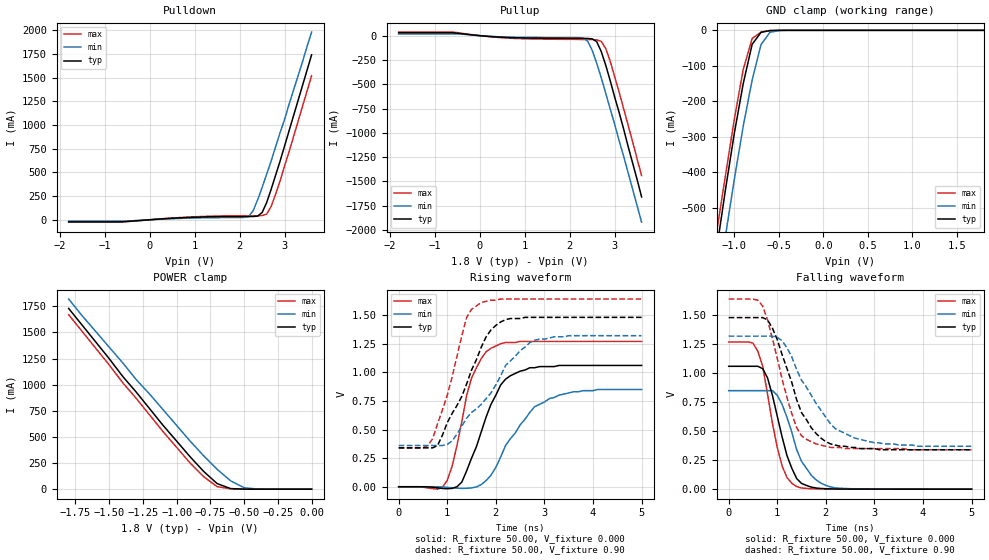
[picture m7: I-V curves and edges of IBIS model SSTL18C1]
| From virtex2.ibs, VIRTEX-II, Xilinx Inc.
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|   Model SSTL18C1
[Model]   SSTL18C1
Model_type   I/O
Polarity   Non-Inverting
Enable   Active-Low
Vinh = 1.025v
Vinl = 0.775v
Vmeas =   0.90V
Cref =  30.00pF
Rref =  50.00
Vref =   0.90V
C_comp   7.00pF   6.00pF   8.00pF
[Temperature Range]   25.00   100.00   0.000
[Voltage Range]   1.80V   1.70V   1.90V
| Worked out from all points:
|   slope of the pulldown table from 0 to 0.27 V, typ, clamps not added: 29.1 ohm
|   slope of the pullup table from 0 to 0.27 V, typ, clamps not added: 26.6 ohm
|   GND clamp passes 1 mA (typ) near -0.61 V on its own axis
|   POWER clamp passes 1 mA (typ) near -0.51 V on its own axis
|   rising waveform, R_fixture 50.00, V_fixture 0.000: 20-80 % time 588ps typ, 760ps min, 432ps max; typ from 0 V to 1.06 V
|   rising waveform, R_fixture 50.00, V_fixture 0.90: 20-80 % time 726ps typ, 1.04ns min, 496ps max; typ from 0.34 V to 1.48 V
|   falling waveform, R_fixture 50.00, V_fixture 0.000: 20-80 % time 396ps typ, 471ps min, 348ps max; typ from 1.06 V to 0 V
|   falling waveform, R_fixture 50.00, V_fixture 0.90: 20-80 % time 616ps typ, 791ps min, 492ps max; typ from 1.48 V to 0.34 V
[Pulldown]
| voltage   I(typ)   I(min)   I(max)
-1.8V     -22.43mA   -14.43mA   -25.5mA
-700mV    -22.43mA   -14.43mA   -25.5mA
900mV     24.93mA    17.53mA    29.31mA
2.2V      34.25mA    34.8mA     41.86mA
2.3V      34.66mA    95.09mA    41.97mA
2.4V      38.31mA    210mA      42.34mA
2.5V      76.54mA    340mA      44.73mA
2.6V      180mA      480mA      59.03mA
2.7V      320mA      620mA      140mA
2.9V      620mA      920mA      410mA
3V        780mA      1.06A      570mA
3.6V      1.74A      1.98A      1.52A
[Pullup]
| voltage   I(typ)   I(min)   I(max)
-1.8V     29.35mA    17.06mA    36.57mA
-600mV    29.35mA    17.06mA    36.57mA
600mV     -18.84mA   -14.55mA   -24.59mA
2.2V      -28.12mA   -21.34mA   -38.85mA
2.4V      -29.08mA   -55.84mA   -39.41mA
2.5V      -33.23mA   -150mA     -40.04mA
2.6V      -60.46mA   -280mA     -43.55mA
2.7V      -160mA     -430mA     -57.58mA
2.8V      -300mA     -590mA     -130mA
2.9V      -460mA     -750mA     -260mA
3.1V      -790mA     -1.08A     -580mA
3.6V      -1.66A     -1.92A     -1.44A
[GND_clamp]
| voltage   I(typ)   I(min)   I(max)
-1.8V     -1.65A     -1.74A     -1.6A
-1.2V     -620mA     -740mA     -570mA
-1.1V     -450mA     -580mA     -410mA
-1V       -290mA     -420mA     -250mA
-900mV    -150mA     -270mA     -110mA
-800mV    -39.2mA    -140mA     -23mA
-700mV    -5.61mA    -40.17mA   -4.8mA
-600mV    -750uA     -5.57mA    -620uA
-500mV    -57.3uA    -660uA     -36.33uA
1.8V      30.92pA    98.88nA    20.22pA
[POWER_clamp]
| voltage   I(typ)   I(min)   I(max)
-1.8V     1.73A      1.82A      1.67A
-1.7V     1.57A      1.66A      1.51A
-1.4V     1.08A      1.21A      1.02A
-1.3V     930mA      1.05A      870mA
-1.1V     610mA      760mA      550mA
-900mV    310mA      460mA      250mA
-800mV    170mA      320mA      120mA
-700mV    53.56mA    190mA      24.17mA
-600mV    5.5mA      79.88mA    3.5mA
-500mV    490uA      13.45mA    470uA
-400mV    34.21uA    820uA      28.36uA
0V        30.92pA    1.07nA     28.99pA
[Ramp]
| variable   typ   min   max
dV/dt_r   0.64/0.57n   0.51/0.80n   0.76/0.43n
dV/dt_f   0.64/0.76n   0.50/1.09n   0.72/0.59n
R_load = 50.00
[Rising Waveform]
R_fixture = 50.00
V_fixture = 0.000
| time   V(typ)   V(min)   V(max)
0s        0V         0V         0V
800ps     -9.52mV    -300uV     -21.25mV
1ns       -17.24mV   -5.02mV    56.09mV
1.3ns     40.76mV    -14.5mV    570mV
1.5ns     250mV      -9.9mV     950mV
1.9ns     720mV      100mV      1.21V
2.2ns     940mV      360mV      1.26V
2.8ns     1.04V      700mV      1.27V
3.6ns     1.06V      830mV      1.27V
5ns       1.06V      850mV      1.27V
[Rising Waveform]
R_fixture = 50.00
V_fixture = 0.90
V_fixture_min = 0.79
V_fixture_max = 1.01
| time   V(typ)   V(min)   V(max)
0s        340mV      360mV      340mV
500ps     340mV      360mV      340mV
700ps     340mV      360mV      420mV
800ps     360mV      360mV      550mV
1.1ns     640mV      400mV      960mV
1.4ns     900mV      600mV      1.48V
1.7ns     1.22V      720mV      1.61V
2.1ns     1.44V      970mV      1.64V
2.8ns     1.48V      1.28V      1.64V
5ns       1.48V      1.32V      1.64V
[Falling Waveform]
R_fixture = 50.00
V_fixture = 0.000
| time   V(typ)   V(min)   V(max)
0s        1.06V      850mV      1.27V
500ps     1.06V      850mV      1.26V
700ps     1.04V      850mV      1.06V
800ps     960mV      850mV      820mV
1ns       630mV      810mV      360mV
1.1ns     450mV      730mV      200mV
1.4ns     91.35mV    340mV      22.19mV
1.7ns     17.79mV    120mV      3.93mV
2.1ns     2.31mV     18.83mV    1.06mV
5ns       21.01uV    110uV      3.42uV
[Falling Waveform]
R_fixture = 50.00
V_fixture = 0.90
V_fixture_min = 0.79
V_fixture_max = 1.01
| time   V(typ)   V(min)   V(max)
0s        1.48V      1.32V      1.64V
700ps     1.48V      1.32V      1.58V
900ps     1.39V      1.32V      1.3V
1.1ns     1.16V      1.28V      950mV
1.3ns     920mV      1.14V      650mV
1.4ns     770mV      1.03V      530mV
1.6ns     600mV      880mV      430mV
2.1ns     390mV      560mV      360mV
2.6ns     360mV      440mV      350mV
5ns       340mV      370mV      340mV
